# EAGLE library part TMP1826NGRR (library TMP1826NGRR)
Board Mount Temperature Sensors 1-Wire +/-0.2C accurate digital temperature sensor with 2-kbit EEPROM Source: Datasheet
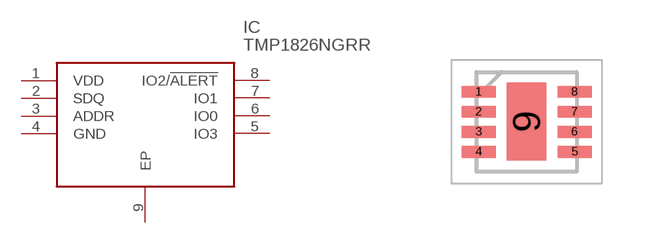
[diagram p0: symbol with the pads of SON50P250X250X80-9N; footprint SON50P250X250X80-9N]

Designator prefix IC

## TMP1826NGRR (Description: Board Mount Temperature Sensors 1-Wire +/-0.2C accurate digital temperature sensor with 2-kbit EEPROM; Height: 0.8mm; Manufacturer_Name: Texas Instruments; Manufacturer_Part_Number: TMP1826NGRR; Mouser_Part_Number: 595-TMP1826NGRR; Mouser_Price-Stock: https://www.mouser.co.uk/ProductDetail/Texas-Instruments/TMP1826NGRR?qs=11PymoJGorLoOZ7sctxtgw%3D%3D)  [SON50P250X250X80-9N]
1  VDD
2  SDQ
3  ADDR
4  GND
5  IO3
6  IO0
7  IO1
8  IO2/!ALERT
9  EP

## Footprint SON50P250X250X80-9N (pad centres in mm)
NGR0008C
smd 0.85 x 0.3: 1 -1.2,0.75; 2 -1.2,0.25; 3 -1.2,-0.25; 4 -1.2,-0.75; 5 1.2,-0.75; 6 1.2,-0.25; 7 1.2,0.25; 8 1.2,0.75
smd 0.98 x 1.95: 9 0,0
